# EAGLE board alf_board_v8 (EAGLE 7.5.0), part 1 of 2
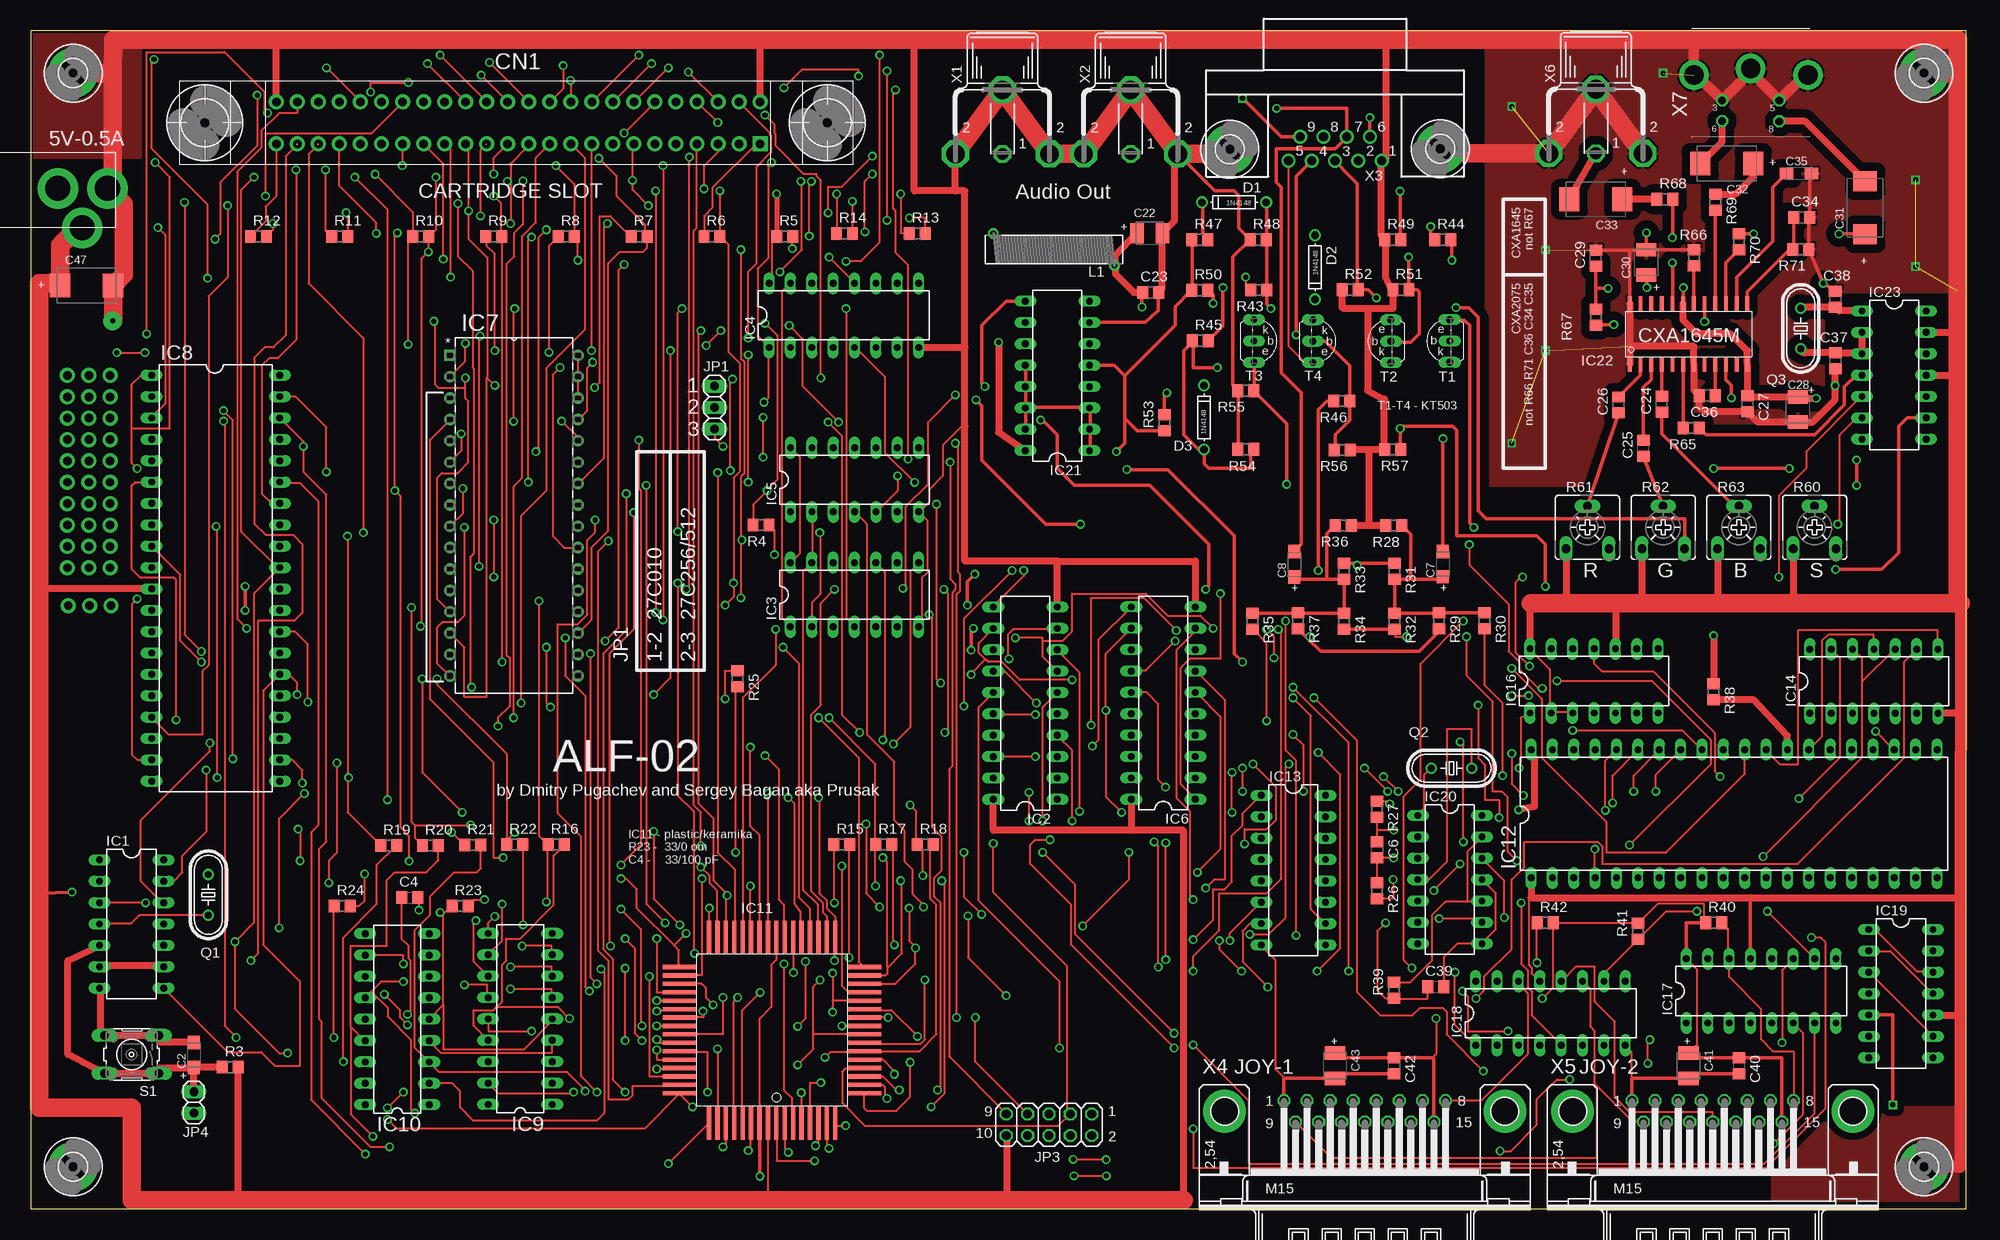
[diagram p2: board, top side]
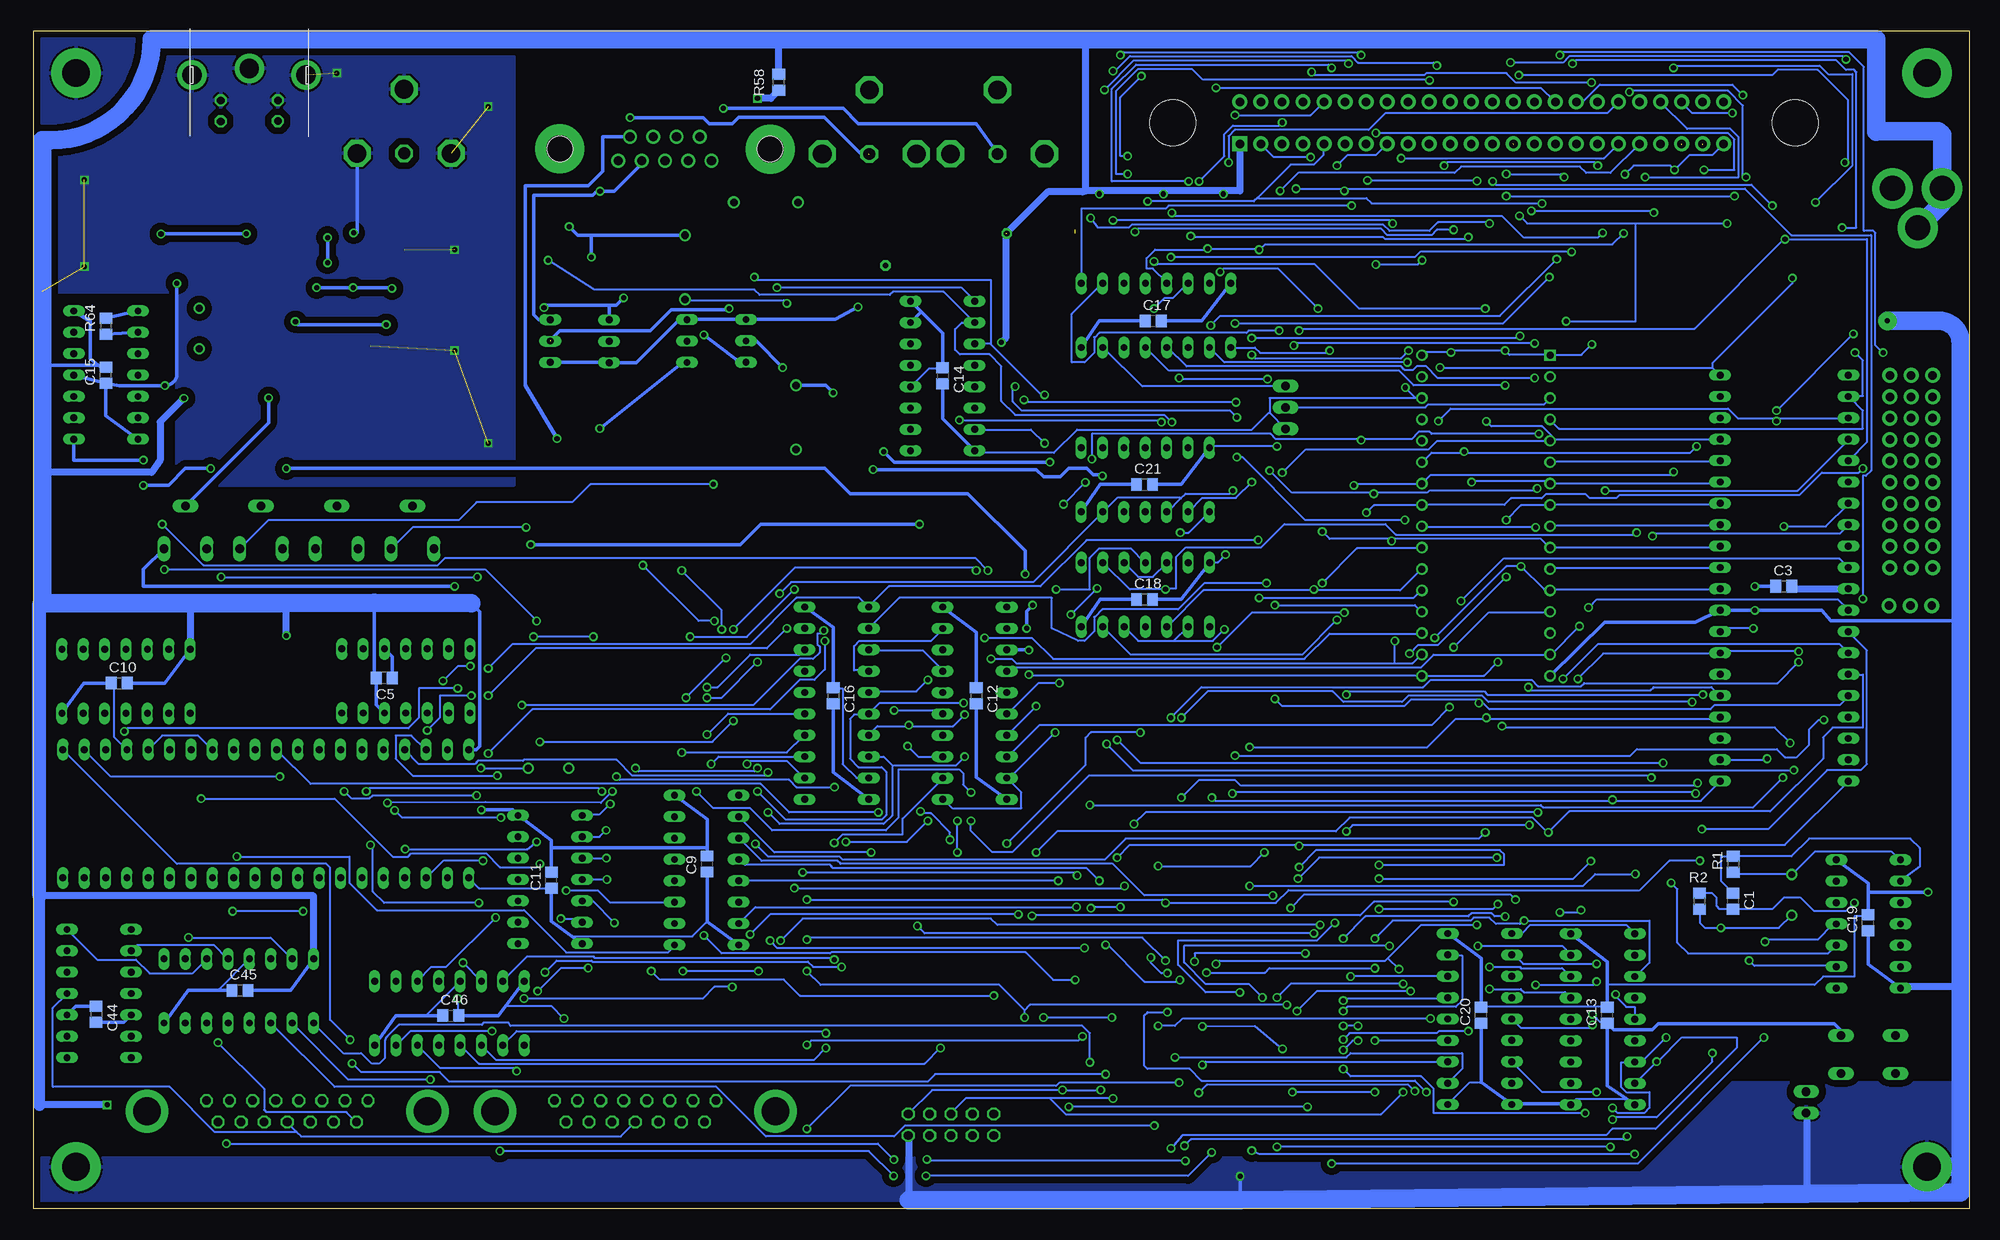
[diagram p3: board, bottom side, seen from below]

Size 230 x 140 mm. Coordinates in mm from the lower left corner, seen from the top.
Outline: 0,0 230,0 230,140 0,140 0,0
Copper layers (1*16): Top 0.035mm / dielectric 1.5mm / Bottom 0.035mm
Design rules "default *": minimum track width 10mil, minimum drill 24mil, track to track 8mil, track to pad 8mil, pad to pad 8mil, via to via 8mil, smd to smd 8mil, copper to edge 4mil, drill to drill 8mil, minimum pad ring 10mil, minimum via ring 8mil, stop-mask expansion 4mil, vias tented up to drill 24mil, thermal gap 10mil

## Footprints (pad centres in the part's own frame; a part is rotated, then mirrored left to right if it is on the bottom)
C0805 = smd 1.3 x 1.5: 1 -0.95,0; 2 0.95,0
SMC_A = smd 1.6 x 1.4: + -1.5,0; - 1.5,0
SMC_B = smd 1.6 x 2.4: + -1.5,0; - 1.5,0
SMC_D = smd 2.4 x 2.8: + -3.15,0; - 3.15,0
СНП15-48 = drill 1 pad 1.778 square: 1 29,-2.5 | drill 1 pad 1.778: 2 29,2.5; 3 26.5,-2.5; 4 26.5,2.5; 5 24,-2.5; 6 24,2.5; 7 21.5,-2.5; 8 21.5,2.5; 9 19,-2.5; 10 19,2.5; 11 16.5,-2.5; 12 16.5,2.5; 13 14,-2.5; 14 14,2.5; 15 11.5,-2.5; 16 11.5,2.5; 17 9,-2.5; 18 9,2.5; 19 6.5,-2.5; 20 6.5,2.5; 21 4,-2.5; 22 4,2.5; 23 1.5,-2.5; 24 1.5,2.5; 25 -1,-2.5; 26 -1,2.5; 27 -3.5,-2.5; 28 -3.5,2.5; 29 -6,-2.5; 30 -6,2.5; 31 -8.5,-2.5; 32 -8.5,2.5; 33 -11,-2.5; 34 -11,2.5; 35 -13.5,-2.5; 36 -13.5,2.5; 37 -16,-2.5; 38 -16,2.5; 39 -18.5,-2.5; 40 -18.5,2.5; 41 -21,-2.5; 42 -21,2.5; 43 -23.5,-2.5; 44 -23.5,2.5; 45 -26,-2.5; 46 -26,2.5; 47 -28.5,-2.5; 48 -28.5,2.5
DO-1N4148 = drill 0.9: A -3.81,0; C 3.81,0
3,3-PAD = drill 3.3 pad 5.842: B3,3 0,0
3,2-PAD = drill 3.2 pad 5.842: B3,2 0,0
DIL14 = drill 0.813 long: 1 -7.62,-3.81; 2 -5.08,-3.81; 3 -2.54,-3.81; 4 0,-3.81; 5 2.54,-3.81; 6 5.08,-3.81; 7 7.62,-3.81; 8 7.62,3.81; 9 5.08,3.81; 10 2.54,3.81; 11 0,3.81; 12 -2.54,3.81; 13 -5.08,3.81; 14 -7.62,3.81
DIL20 = drill 0.813 long: 1 -11.43,-3.81; 2 -8.89,-3.81; 3 -6.35,-3.81; 4 -3.81,-3.81; 5 -1.27,-3.81; 6 1.27,-3.81; 7 3.81,-3.81; 8 6.35,-3.81; 9 8.89,-3.81; 10 11.43,-3.81; 11 11.43,3.81; 12 8.89,3.81; 13 6.35,3.81; 14 3.81,3.81; 15 1.27,3.81; 16 -1.27,3.81; 17 -3.81,3.81; 18 -6.35,3.81; 19 -8.89,3.81; 20 -11.43,3.81
DIL16 = drill 0.813 long: 1 -8.89,-3.81; 2 -6.35,-3.81; 3 -3.81,-3.81; 4 -1.27,-3.81; 5 1.27,-3.81; 6 3.81,-3.81; 7 6.35,-3.81; 8 8.89,-3.81; 9 8.89,3.81; 10 6.35,3.81; 11 3.81,3.81; 12 1.27,3.81; 13 -1.27,3.81; 14 -3.81,3.81; 15 -6.35,3.81; 16 -8.89,3.81
DIP254P1524X482-32P = drill 0.838 square: 1 -15.24,38.1 | drill 0.838: 2 -15.24,35.56; 3 -15.24,33.02; 4 -15.24,30.48; 5 -15.24,27.94; 6 -15.24,25.4; 7 -15.24,22.86; 8 -15.24,20.32; 9 -15.24,17.78; 10 -15.24,15.24; 11 -15.24,12.7; 12 -15.24,10.16; 13 -15.24,7.62; 14 -15.24,5.08; 15 -15.24,2.54; 16 -15.24,0; 17 0,0; 18 0,2.54; 19 0,5.08; 20 0,7.62; 21 0,10.16; 22 0,12.7; 23 0,15.24; 24 0,17.78; 25 0,20.32; 26 0,22.86; 27 0,25.4; 28 0,27.94; 29 0,30.48; 30 0,33.02; 31 0,35.56; 32 0,38.1
DIL40 = drill 0.813 long: 1 -24.13,-7.62; 2 -21.59,-7.62; 3 -19.05,-7.62; 4 -16.51,-7.62; 5 -13.97,-7.62; 6 -11.43,-7.62; 7 -8.89,-7.62; 8 -6.35,-7.62; 9 -3.81,-7.62; 10 -1.27,-7.62; 11 1.27,-7.62; 12 3.81,-7.62; 13 6.35,-7.62; 14 8.89,-7.62; 15 11.43,-7.62; 16 13.97,-7.62; 17 16.51,-7.62; 18 19.05,-7.62; 19 21.59,-7.62; 20 24.13,-7.62; 21 24.13,7.62; 22 21.59,7.62; 23 19.05,7.62; 24 16.51,7.62; 25 13.97,7.62; 26 11.43,7.62; 27 8.89,7.62; 28 6.35,7.62; 29 3.81,7.62; 30 1.27,7.62; 31 -1.27,7.62; 32 -3.81,7.62; 33 -6.35,7.62; 34 -8.89,7.62; 35 -11.43,7.62; 36 -13.97,7.62; 37 -16.51,7.62; 38 -19.05,7.62; 39 -21.59,7.62; 40 -24.13,7.62
DIL18 = drill 0.813 long: 1 -10.16,-3.81; 2 -7.62,-3.81; 3 -5.08,-3.81; 4 -2.54,-3.81; 5 0,-3.81; 6 2.54,-3.81; 7 5.08,-3.81; 8 7.62,-3.81; 9 10.16,-3.81; 10 10.16,3.81; 11 7.62,3.81; 12 5.08,3.81; 13 2.54,3.81; 14 0,3.81; 15 -2.54,3.81; 16 -5.08,3.81; 17 -7.62,3.81; 18 -10.16,3.81
TQFP64 = smd 0.5 x 4: 1 -1.5,-13; 2 -0.5,-13; 3 0.5,-13; 4 1.5,-13; 5 2.5,-13; 6 3.5,-13; 7 4.5,-13; 8 5.5,-13; 25 5.5,9; 26 4.5,9; 27 3.5,9; 28 2.5,9; 29 1.5,9; 30 0.5,9; 31 -0.5,9; 32 -1.5,9; 33 -2.5,9; 34 -3.5,9; 35 -4.5,9; 36 -5.5,9; 37 -6.5,9; 38 -7.5,9; 39 -8.5,9; 40 -9.5,9; 57 -9.5,-13; 58 -8.5,-13; 59 -7.5,-13; 60 -6.5,-13; 61 -5.5,-13; 62 -4.5,-13; 63 -3.5,-13; 64 -2.5,-13 | smd 4 x 0.5: 9 9,-9.5; 10 9,-8.5; 11 9,-7.5; 12 9,-6.5; 13 9,-5.5; 14 9,-4.5; 15 9,-3.5; 16 9,-2.5; 17 9,-1.5; 18 9,-0.5; 19 9,0.5; 20 9,1.5; 21 9,2.5; 22 9,3.5; 23 9,4.5; 24 9,5.5; 41 -13,5.5; 42 -13,4.5; 43 -13,3.5; 44 -13,2.5; 45 -13,1.5; 46 -13,0.5; 47 -13,-0.5; 48 -13,-1.5; 49 -13,-2.5; 50 -13,-3.5; 51 -13,-4.5; 52 -13,-5.5; 53 -13,-6.5; 54 -13,-7.5; 55 -13,-8.5; 56 -13,-9.5
SOP24 = smd 0.45 x 1.8: 1 -6.97,-3.6; 2 -5.7,-3.6; 3 -4.43,-3.6; 4 -3.16,-3.6; 5 -1.89,-3.6; 6 -0.62,-3.6; 7 0.65,-3.6; 8 1.92,-3.6; 9 3.19,-3.6; 10 4.46,-3.6; 11 5.73,-3.6; 12 7,-3.6; 13 7,3.6; 14 5.73,3.6; 15 4.46,3.6; 16 3.19,3.6; 17 1.92,3.6; 18 0.65,3.6; 19 -0.62,3.6; 20 -1.89,3.6; 21 -3.16,3.6; 22 -4.43,3.6; 23 -5.7,3.6; 24 -6.97,3.6
PJ-102A = drill 3 pad 4.8: RING 0.1,-3.39; RING_SW -4.6,-6.29; TIP 0.1,-9.29
1X03 = drill 1.016 long: 1 -2.54,0; 2 0,0; 3 2.54,0
2X05 = drill 1.016 octagon: 1 -5.08,-1.27; 2 -5.08,1.27; 3 -2.54,-1.27; 4 -2.54,1.27; 5 0,-1.27; 6 0,1.27; 7 2.54,-1.27; 8 2.54,1.27; 9 5.08,-1.27; 10 5.08,1.27
1X02 = drill 1.016 long: 1 -1.27,0; 2 1.27,0
Z27/24 = drill 0.7 octagon: 1 7.2,-1.9; 2 -7.2,1.9
HC49/S = drill 0.813: 1 -2.413,0; 2 2.413,0
R0805 = smd 1.3 x 1.5: 1 -0.95,0; 2 0.95,0
CA6V = drill 1.016 long: A -2.54,-2.54; E 2.54,-2.54; S 0,2.54
B3F-10XX = drill 1.016 long: 1 -3.251,2.261; 2 3.251,2.261; 3 -3.251,-2.261; 4 3.251,-2.261
TO92-CBE = drill 0.813 long: B 0,0; C -2.54,0; E 2.54,0
5,5 = hole 5.5: 0,0
TOBU3 = drill 1.397 octagon: 1 0,-2.54 | drill 2.21 octagon: 2 5.588,-2.54; 2@1 -5.588,-2.54; 2@2 0,5.08
H5M09RA = drill 1.092: 1 -5.537,1.422; 2 -2.769,1.422; 3 0,1.422; 4 2.769,1.422; 5 5.537,1.422; 6 -4.153,-1.422; 7 -1.384,-1.422; 8 1.384,-1.422; 9 4.153,-1.422 | hole 3.048: -12.497,0; 12.497,0
M15HP = drill 1.016 octagon: 1 -9.601,1.27; 2 -6.858,1.27; 3 -4.115,1.27; 4 -1.372,1.27; 5 1.372,1.27; 6 4.115,1.27; 7 6.858,1.27; 8 9.601,1.27; 9 -8.23,-1.27; 10 -5.486,-1.27; 11 -2.743,-1.27; 12 0,-1.27; 13 2.743,-1.27; 14 5.486,-1.27; 15 8.23,-1.27 | drill 3.302 pad 5.08: G1 -16.662,0; G2 16.662,0
M_DIN4 = drill 0.9 pad 1.422 octagon: 3 -3.4,-3.75; 5 3.4,-3.75; 6 -3.4,-6.2; 8 3.4,-6.25 | drill 2.3 pad 3.5: SH1 6.8,-0.75; SH2 0,0.05; SH3 -6.75,-0.75

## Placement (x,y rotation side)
C1  68pF  [C0805]  28.06,36.58 270 bottom
C2  10uF 16V  [SMC_A]  19.36,18.29 90 top
C3  [C0805]  22,74 0 bottom
C4  33/100pF  [C0805]  45,37 0 top
C5  [C0805]  188.35,63.1 180 bottom
C6  68pF  [C0805]  159.99,42.66 270 top
C7  1uF  [SMC_A]  167.81,76.63 90 top
C8  1uF  [SMC_A]  150.16,76.61 90 top
C9  [C0805]  149.99,40.99 90 bottom
C10  [C0805]  219.86,62.49 0 bottom
C11  [C0805]  168.49,39.04 90 bottom
C12  [C0805]  118,61 270 bottom
C13  [C0805]  43,23 90 bottom
C14  [C0805]  122,99 270 bottom
C15  [C0805]  221.45,99.1 90 bottom
C16  [C0805]  135,61 270 bottom
C17  [C0805]  96.95,105.55 0 bottom
C18  [C0805]  98,72.45 0 bottom
C19  [C0805]  12,34 90 bottom
C20  [C0805]  58,23 90 bottom
C21  [C0805]  98,86.1 0 bottom
C22  100uF  [SMC_B]  132.98,115.97 0 top
C23  [C0805]  133.09,108.94 0 top
C24  [C0805]  193.85,95.65 90 top
C25  [C0805]  191.65,90.4 90 top
C26  [C0805]  188.7,95.55 90 top
C27  [C0805]  204,95.7 270 top
C28  47uF  [SMC_B]  210,95 270 top
C29  [C0805]  186,113 90 top
C30  47uF  [SMC_B]  192,112.5 90 top
C31  220uF  [SMC_D]  218,119 90 top
C32  220uF  [SMC_D]  201.55,124.25 180 top
C33  220uF  [SMC_D]  186,120 180 top
C34  [C0805]  210.45,117.85 0 top
C35  10uF  [SMC_A]  210.15,123.05 0 top
C36  [C0805]  199.25,96.65 180 top
C37  33  [C0805]  214.5,100.8 90 top
C38  33  [C0805]  214.45,108.1 270 top
C39  4n7  [C0805]  166.95,26.4 0 top
C40  [C0805]  203,17 270 top
C41  50uF  [SMC_B]  197,17 270 top
C42  [C0805]  162,17 270 top
C43  50uF  [SMC_B]  155,17 270 top
C44  [C0805]  222.61,23.11 270 bottom
C45  [C0805]  205.51,25.97 0 bottom
C46  [C0805]  180.46,22.97 0 bottom
C47  220uF  [SMC_D]  6.6,109.75 0 top
CN1  СНП15-48  [СНП15-48]  57.66,129.08 0 top
D1  1N4148  [DO-1N4148]  143,119.63 180 top
D2  1N4148  [DO-1N4148]  152.62,111.91 270 top
D3  1N4148  [DO-1N4148]  139.43,94.07 90 top
H1  MOUNT-PAD-ROUND3.3  [3,3-PAD]  5,135 0 top
H2  MOUNT-PAD-ROUND3.3  [3,3-PAD]  225,135 0 top
H3  MOUNT-PAD-ROUND3.3  [3,3-PAD]  225,5 0 top
H4  MOUNT-PAD-ROUND3.3  [3,3-PAD]  5,5 0 top
H5  MOUNT-PAD-ROUND3.2  [3,2-PAD]  142.5,125.95 0 top
H6  MOUNT-PAD-ROUND3.2  [3,2-PAD]  167.5,126 0 top
IC1  LS04/1533LN1  [DIL14]  11.95,33.86 270 top
IC2  ALS240 / 1533AP3  [DIL20]  118.18,60.1 90 top
IC3  ALS32/1533LL1  [DIL14]  97.88,73 0 top
IC4  ALS175/1533TM8  [DIL16]  96.62,106.2 0 top
IC5  ALS09/1533LI2  [DIL14]  97.9,86.65 0 top
IC6  LS245 / 555AP6  [DIL20]  134.58,60.11 90 top
IC7  27C010  [DIP254P1524X482-32P]  65.03,63.35 0 top
IC8  Z80A  [DIL40]  21.96,74.96 270 top
IC9  41464/RU11  [DIL18]  58.15,22.57 90 top
IC10  41464/RU11  [DIL18]  43.53,22.54 90 top
IC11  T34VG1  [TQFP64]  90.09,23.24 0 top
IC12  YM2149F / AY-3-8910  [DIL40]  202.43,46.96 0 top
IC13  ALS138/1533ID7  [DIL16]  150.05,40.26 270 top
IC14  ALS00/1533LA3  [DIL14]  219.05,62.7 0 top
IC16  ALS93/1533IE5  [DIL14]  185.79,62.75 0 top
IC17  74HC595  [DIL16]  205.65,25.9 0 top
IC18  74HC595  [DIL16]  180.61,23.25 0 top
IC19  7493 / 155IE5  [DIL14]  222.26,25.59 270 top
IC20  ALS04/1533LN1  [DIL14]  168.65,39.14 270 top
IC21  ALS251/1533KP15  [DIL16]  122,99 90 top
IC22  CXA1645  [SOP24]  197,104 0 top
IC23  74HCT04  [DIL14]  221.45,99.1 270 top
J1  2.1MMJACKTHM  [PJ-102A]  -0.2,121.2 90 top
JP1  [1X03]  81.25,95.25 270 top
JP3  V-TTL-OUT  [2X05]  121,10 180 top
JP4  RESET  [1X02]  19.35,12.65 270 top
L1  220 uH  [Z27/24]  121.59,114.03 180 top
Q1  8Mhz  [HC49/S]  21.08,37.33 270 top
Q2  14Mhz  [HC49/S]  168.84,52.38 0 top
Q3  4,433619Mhz  [HC49/S]  210.35,104.65 270 top
R1  510  [R0805]  28.02,40.95 90 bottom
R2  510  [R0805]  32.03,36.58 270 bottom
R3  100k  [R0805]  23.69,16.84 0 top
R4  1.6k  [R0805]  86.77,81.28 180 top
R5  2.2k  [R0805]  89.59,115.59 0 top
R6  2.2k  [R0805]  80.94,115.59 0 top
R7  2.2k  [R0805]  72.29,115.59 0 top
R8  2.2k  [R0805]  63.64,115.59 0 top
R9  2.2k  [R0805]  54.99,115.59 0 top
R10  2.2k  [R0805]  46.34,115.59 0 top
R11  2.2k  [R0805]  36.69,115.59 0 top
R12  2.2k  [R0805]  27.04,115.59 0 top
R13  10k  [R0805]  105.34,115.94 0 top
R14  10k  [R0805]  96.69,115.94 0 top
R15  1k  [R0805]  96.39,43.29 0 top
R16  1k  [R0805]  62.44,43.29 0 top
R17  1k  [R0805]  101.36,43.29 0 top
R18  1k  [R0805]  106.29,43.29 0 top
R19  1k  [R0805]  42.5,43.19 0 top
R20  1k  [R0805]  47.48,43.19 0 top
R21  1k  [R0805]  52.51,43.24 0 top
R22  1k  [R0805]  57.49,43.29 0 top
R23  33/0  [R0805]  51,36 0 top
R24  33  [R0805]  37,36 0 top
R25  300  [R0805]  83.99,63.02 270 top
R26  510  [R0805]  159.97,37.81 270 top
R27  510  [R0805]  159.97,47.51 270 top
R28  2.2k  [R0805]  161.99,81.22 0 top
R29  1k  [R0805]  167.35,69.9 270 top
R30  1k  [R0805]  172.77,69.91 270 top
R31  15k  [R0805]  162.07,75.81 270 top
R32  2.2k  [R0805]  162.07,69.86 270 top
R33  15k  [R0805]  156.07,75.81 270 top
R34  2.2k  [R0805]  156.07,69.86 270 top
R35  1k  [R0805]  145.17,69.86 270 top
R36  2.2k  [R0805]  155.96,81.23 180 top
R37  1k  [R0805]  150.6,69.9 270 top
R38  1k  [R0805]  199.99,61.46 270 top
R39  1.5k  [R0805]  162,26 90 top
R40  10k  [R0805]  200,34 0 top
R41  1k  [R0805]  191.01,32.99 90 top
R42  10k  [R0805]  180,34 0 top
R43  1k  [R0805]  145.91,109.21 180 top
R44  1k  [R0805]  167.79,115.19 0 top
R45  1k  [R0805]  138.99,103.19 0 top
R46  1.5k  [R0805]  155.81,96.01 180 top
R47  3k3  [R0805]  138.94,115.19 0 top
R48  3k3  [R0805]  145.89,115.19 0 top
R49  200  [R0805]  161.84,115.19 0 top
R50  3k3  [R0805]  138.94,109.19 0 top
R51  3k3  [R0805]  162.84,109.24 0 top
R52  200  [R0805]  156.79,109.24 0 top
R53  3k3  [R0805]  134.71,93.44 90 top
R54  3k3  [R0805]  144.39,90.29 0 top
R55  200  [R0805]  144.39,97.24 0 top
R56  2k  [R0805]  155.86,90.21 180 top
R57  200  [R0805]  161.84,90.24 0 top
R58  100  [R0805]  141.47,133.89 90 bottom
R60  [CA6V]  212,81 0 top
R61  [CA6V]  185,81 0 top
R62  [CA6V]  194,81 0 top
R63  [CA6V]  203,81 0 top
R64  4.7M  [R0805]  221.45,104.9 90 bottom
R65  1.6k  [R0805]  197.35,92.8 180 top
R66  16k  [R0805]  197.65,113.05 90 top
R67  2.4k  [R0805]  186,106 270 top
R68  75  [R0805]  194.2,120 0 top
R69  75  [R0805]  200.2,119.65 270 top
R70  75  [R0805]  203,114.95 270 top
R71  47k  [R0805]  210.35,114.05 180 top
S1  RESET  [B3F-10XX]  11.97,18.35 180 top
T1  [TO92-CBE]  168.63,103.15 90 top
T2  [TO92-CBE]  161.63,103.12 90 top
T3  [TO92-CBE]  145.37,103.16 270 top
T4  [TO92-CBE]  152.37,103.14 270 top
U$2  [5,5]  20.65,129.1 0 top
U$3  [5,5]  94.65,129.1 0 top
X1  RCA_L  [TOBU3]  115.47,127.93 0 top
X2  RCA_R  [TOBU3]  130.71,127.93 0 top
X3  RGB-OUT  [H5M09RA]  155,126 180 top
X4  JOY-1  [M15HP]  158.53,11.59 0 top
X5  JOY-2  [M15HP]  199.89,11.59 0 top
X6  Video  [TOBU3]  186,128 0 top
X7  s-video  [M_DIN4]  204.4,135.5 0 top

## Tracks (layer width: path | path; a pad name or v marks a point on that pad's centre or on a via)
1IC8  (via drill 0.61)
  Top 0.254: v141.38,73.12 141.38,65.38 137.75,65.38 136.62,64.25 136.62,50.5 138.38,48.75 IC6.1 | v49.88,110.75 49.88,125.88 49.25,126.5 CN1.31 | v87.25,105.25 88.75,103.75 88.75,86.75 87.5,85.5 v87.5,85.38 85.82,83.69 R4.2
  Bottom 0.254: v87.5,85.38 87.88,85 93.12,85 93.69,84.44 | 93.69,84.44 95.25,82.88 IC5.3 | 93.69,84.44 93.75,84.5 101.25,84.5 102.88,82.88 IC5.6 103,82.75 111.25,74.5 140,74.5 v141.38,73.12 | v49.88,110.75 55.38,105.25 v87.25,105.25
8M  (via drill 0.61)
  Top 0.254: IC1.4 8.25,33.88 11.88,33.88 12.88,34.88 21,34.88 Q1.2 | v87.55,49.38 87.55,32.5 87.5,32.25 IC11.33 | v32.5,49.38 29.5,46.38 v29.5,33.4
  Bottom 0.254: v87.55,49.38 87.12,49.5 32.62,49.5 v32.5,49.38 | R2.2 32,35.6 32,34 31.4,33.4 v29.5,33.4 22.6,33.4 Q1.2
+5V  (via drill 0.6, 0.6 pad 0.25, 0.61)  (1 unrouted)
  Top 0.254: IC3.14 90.38,76.88 91.38,77.88 91.38,89.38 90.38,90.38 IC5.14 | v67,97.62 67.62,98.25 67.62,118 68.88,118 71.25,115.62 R7.1 | v82.25,90.62 81.25,91.62 JP1.3 | R12.1 27.88,117.38 27.88,119.12 29.12,120.38 29.12,126.5 CN1.47 | v35,123.5 35,116.25 35.62,115.62 R11.1 | 45.38,115.62 R10.1 | v55.12,102 55.12,113.5 54.12,114.5 54.12,115.5 R9.1 | 62.62,115.5 R8.1 61.58,114.47 v61.58,101.8 | IC7.32 65,101.38 65,99 IC7.31 65,98.88 65,96.38 IC7.30 | 45.5,115.5 R10.1 | IC4.16 87.75,110.12 88.12,110.5 88.12,115 88.62,115.5 R5.1 88.62,115.62 | 24.62,16.75 R3.2 | 200,62.5 R38.1 | 80,115.62 R6.1 80,118 81,119 81,121.38 86.12,126.5 86.62,126.5 CN1.1 | v95.75,120.62 95.75,116 R14.1 | v103.38,120.62 103.38,116 R13.1 | 87.62,1 87.62,10.12 IC11.64 | R40.1 198.88,34.12 198.88,36.25 193.38,36.25 191.12,34 R41.2 191,34 R42.2 180.88,34 180.88,26.25 v179.62,25 | v167,22.62 167,18.38 166.75,18.12 166.75,17.95 | v88.38,77.75 88.38,80.62 R4.1 | v44.83,102.75 44.83,115.03 R10.1 | v40.9,122.97 45.39,118.48 R10.1 | C41.+ 198.05,19.55 198.05,28.42 IC17.16
  Top 0.406: R67.1 186,109.4 | 186,109.4 C29.1 | C30.+ 192.05,111 v192.05,109.5 | v187.45,109.4 186,109.4 | v196.4,109.5 196.38,109.5 IC22.19 | C27.1 204.15,96.5 | R40.1 196.76,34 IC17.16 | C43.+ 155,17.95 C42.1 166.75,17.95 166.76,17.95 X4.15 | C41.+ 197,17.95 C40.1 208.12,17.95 X5.15 | JP3.10 116,8.73 | 1,73.69 1,74 | v4.88,37.65 1,37.5 | IC19.5 221.3,23.05 v221.3,12.35
  Top 0.61: v88.62,120.62 88.62,115.62
  Top 0.813: IC22.19 196.38,105.62 198,104 202,104 204,102 IC22.12 C27.1 | 204.15,96.5 C28.+ 210.15,96.35 v212.2,96.35 | 137,1 137,45 130.77,45 | 130.77,45 114.4,45 114.4,48.67 IC2.20 | IC6.20 130.77,45 | 116,8.73 116,1 | IC8.11 1,73.69 | 24.62,1 24.62,16.75 | v200,68.12 200,62.5 | v176.82,47.42 178.7,47.8 178.7,53.55 IC12.40 | v115,103 115,92.3 IC21.16 | 0.99,47 1,47
  Top 2.184: 137,1 116,1 87.62,1 24.62,1 12,1 12,12 1,12 1,37.5 1,47 1,74 1,110 3.45,110 C47.+ 3.45,114.55 5.5,116.6 J1.RING_SW
  Bottom 0.254: v88.38,77.75 89.25,76.88 90.12,76.88 IC3.14 | 65.81,96.44 65.75,96.38 65.12,96.38 IC7.30 | 65.81,96.44 v67,97.62 | 83.12,94.62 81.25,92.75 JP1.3 | 83.12,94.62 83.12,96.38 65.88,96.38 65.81,96.44 | v82.25,90.62 90,90.62 90.12,90.5 IC5.14 | CN1.47 29.25,126.5 30.5,125.25 33.25,125.25 v35,123.5 35.5,124 39.88,124 v40.9,122.97 | C20.2 57.88,24 43.12,24 C13.2 | v95.75,120.62 95.75,121 | v103.38,120.62 103.38,121 | 114.38,116 L1.1 | v88.62,120.62 88.62,121 | 189.57,63.3 C5.2 | v179.62,25 179.62,23.12 C46.2 | 43,26.62 18.35,26.62 17.32,27.6 13.62,27.6 13.62,34.75 12,34.75 C19.2 | 172.62,46.88 IC20.14 | v167,22.62 168.5,24.12 173.75,24.12 173.87,24.21 | 83.12,94.62 83.25,94.62 85.25,92.62 106,92.62 108.78,89.85 117.93,89.85 arc90 IC21.16 118,90.12 | v44.83,102.75 46.08,101.5 49.75,101.5 IC7.1 49.88,101.5 54.62,101.5 v55.12,102 61.38,102 v61.58,101.8 64.68,101.8 IC7.32
  Bottom 0.406: C19.2 12,37.65 | 12,37.65 12,38.72 IC1.14 | C13.2 43,26.62 43,29.36 IC10.9 | C20.2 58,29.77 IC9.9 | C12.2 118,51.3 IC2.20 | C16.2 135,51.91 IC6.20 | C18.2 93.62,72.45 IC3.14 | C21.2 93.64,86.1 IC5.14 | C17.2 91.19,105.55 IC4.16 | C14.2 122,93.92 IC21.16 | C9.2 149.99,42.9 | 149.99,42.9 149.99,46.28 IC13.16 | C46.2 174.81,22.97 173.87,24.21 IC18.16 | C45.2 199.5,25.97 IC17.16 | C44.2 219.34,22.16 IC19.5 | C10.2 214.45,62.49 IC14.14 211.35,66.59 | C5.2 189.3,59.91 IC16.5 | C11.2 168.49,42.9 | 168.49,42.9 168.49,43.79 IC20.14 | IC23.14 223.3,105.51 223.3,101.05 222.05,100.05 C15.2 221.7,100.3 229,100.3 | v187.45,109.4 187.45,109.5 v192.05,109.5 v196.4,109.5 | 178,72 177,71 177,55 177.42,54.58 IC12.40 | 149.99,42.9 168.49,42.9 | 189.57,72.05 189.57,63.3 | v4.88,37.65 12,37.65 | 172.62,46.88 173.07,47.42 v176.82,47.42 | 141.47,138.47 142,139
  Bottom 0.813: 211.35,66.59 211.35,72 | v212.2,96.35 215,93.55 215,89 216,87.55 229,87.55 | CN1.1 86.66,121 88.62,121 95.75,121 103.38,121 105,121 | 105,121 105,139 | IC17.16 196.76,37.2 229.35,37.2 | v200,68.12 200,72 | 114.38,116 109.5,120.88 105.38,120.88 105,121 | v221.3,12.35 229.35,12.35 | C3.2 20.74,73.69 IC8.11 | R58.2 141.47,138.47 | 114.5,115.88 114.5,103.5 v115,103
  Bottom 1.422: 229.35,12.35 229.35,37.2
  Bottom 1.676: 229.35,37.2 229.35,72 229,72
  Bottom 2.184: 178,72 189.57,72.05 200,72 211.35,72 229,72 229,87.55 229,100.3 229,127 228,127 arc-90 216,139 142,139 105,139 11,139 11,128 10.9,128.1 3.65,128.1 3.19,127.64 J1.RING 3.19,119.5 J1.RING_SW
/BUSRQ  (via drill 0.61)
  Top 0.254: 97.62,116 R14.2 97.62,115.95 v97.62,119.75 | v50.75,119.5 50.75,113.25 52.5,111.5 52.5,100 52.65,99.85 52.65,77.9 52.2,77.45 52.2,62.17 v52.38,62
  Bottom 0.254: v97.62,119.75 85,119.75 84.56,120.19 | 84.56,120.19 80.62,124.12 77.88,124.12 76.75,125.25 76.75,126.5 CN1.9 | v52.38,62 52,61.62 37.88,61.62 37.5,62 30.62,62 29.62,61 IC8.25 | v50.75,119.5 71,119.5 71.62,120.12 84.5,120.12 84.56,120.19
/CAS  (via drill 0.61)
  Top 0.254: v85.5,38.38 85.5,32.25 IC11.35 | R24.2 39,36 39.65,36.65 v39.65,39.8
  Bottom 0.254: v85.5,38.38 45.88,38.38 44.45,39.8 v39.65,39.8
/CE  (via drill 0.61)
  Top 0.254: v93.75,80.38 93.88,80.25 93.88,73.12 92.88,72.12 92.88,69.25 IC3.2 | v88.5,68.88 88.5,64.62 84.62,60.75 84.62,32.25 IC11.36
  Bottom 0.254: 94.44,67.56 94.5,67.5 98.75,67.5 100.38,69.12 IC3.5 | 94.44,67.56 92.88,69.12 IC3.2 | v93.75,80.38 92.75,80.38 90.38,82.75 IC5.1 | v88.5,68.88 89.88,67.5 94.38,67.5 94.44,67.56
/INT  (via drill 0.61)
  Top 0.254: v82.5,60.62 82.5,63.97 R25.1 83.88,63.88 | v58.25,60.12 58.25,82.38 61.25,85.38 61.25,99.9 65.88,104.53 65.88,124.88 64.25,126.5 CN1.19
  Bottom 0.254: v82.5,60.62 81.62,59.75 67.12,59.75 66.38,60.5 58.25,60.5 | 58.25,60.5 58.12,60.5 57,59.38 30.75,59.38 30.25,59.88 15.38,59.88 14.38,60.88 IC8.16 | 58.25,60.5 v58.25,60.12
/IORQ  (via drill 0.61)
  Top 0.254: v103.38,39 103.5,38.88 103.5,30.38 101.81,28.69 | 101.81,28.69 101.81,28.01 101.55,27.75 99.12,27.75 IC11.23 | v101.25,41.75 101.75,41.25 101.75,28.75 101.81,28.69 | v79.62,43.12 79.62,47.12 78.75,48 78.75,116.25 79.12,116.62 79.12,126.5 CN1.7
  Bottom 0.254: v103.38,39 104.88,40.5 135,40.5 135.38,40.88 145.5,40.88 146.12,41.5 IC13.4 | 79.62,43.25 99.75,43.25 v101.25,41.75 | 79.62,43.25 21.88,43.25 14.38,50.75 IC8.20 | v79.62,43.12 79.62,43.25
/M1  (via drill 0.61)
  Top 0.254: v142.5,31.88 142.5,32.75 146.12,36.38 IC13.6 | IC11.22 99.12,26.75 102.75,26.75 105.12,29.12 v105.12,31 105.12,31.12 104.38,31.88 v104.38,35.75 | v20.25,66.25 18.25,68.25 v18.25,119.62 | v35.12,135.62 39.12,131.62 CN1.40 | v100.88,35.88 99.25,37.5 v99.25,45.75 | v51.25,47.12 46.5,51.88 v46.5,63
  Bottom 0.254: v142.5,31.88 141.62,31 v105.12,31 | v20.25,66.25 29.38,66.25 29.5,66.12 IC8.27 29.62,66 43.5,66 v46.5,63 | v18.25,119.62 13.88,124 13.88,134.88 16.75,134.88 17.75,135.88 34.88,135.88 v35.12,135.62 | v104.38,35.75 104.25,35.88 v100.88,35.88 | v99.25,45.75 97.88,47.12 v51.25,47.12
/MREQ  (via drill 0.61)
  Top 0.254: v89.38,66.75 91.25,64.88 91.25,37.05 92.55,35.75 92.55,34.15 92.6,34.15 92.6,34.1 92.5,32.25 IC11.28 | v74.25,121 v74.25,70.88 | v80,121.25 80,124 81.66,125.66 CN1.5 | v12.62,72.5 12,71.88 12,54 12.63,53.37 IC8.19
  Bottom 0.254: v12.62,72.5 12.62,87.12 12.25,87.12 11.62,87.75 11.62,115.75 21.12,115.75 26.62,121.25 74.25,121.25 | v80,121.25 74.25,121.25 | v89.38,66.75 85.25,70.88 v74.25,70.88 | v74.25,121 74.25,121.25
/NMI  (via drill 0.61)  (1 unrouted)
  Top 0.254: 57,122.12 57,124.25 59.12,126.38 59.12,126.5 CN1.23 | 57,122.12 v57,117.12 | v23.38,119.25 23.38,110.75 21.12,108.5 21.12,64.62 20.38,63.88 20.38,56.38 16.38,56.38 14.38,58.38 IC8.17 | 57,122.12 v56.62,122.12 | 106.3,116.35 106.3,117.78 v104.4,117.78
  Bottom 0.254: v104.4,117.78 103.5,116.62 99.88,116.62 99.5,117 69.62,117 68.88,116.25 64.12,116.25 63.12,117.25 57.12,117.25 v57,117.12 | v23.38,119.25 25.88,121.75 56.25,121.75 v56.62,122.12
/RAS  (via drill 0.61)
  Top 0.254: v80.62,35.75 80.62,32.25 IC11.40 | R23.2 52.7,36.75 v53.9,36.75
  Bottom 0.254: v80.62,35.75 79,37.38 54.52,37.38 v53.9,36.75
/RD  (via drill 0.61)
  Top 0.254: v90,48.88 90.75,48.12 90.75,36.27 91.5,35.3 91.5,32.25 IC11.29 | v42.38,48.62 42.38,118.75 v38.5,122.62
  Bottom 0.254: 42.38,48.5 89.62,48.5 v90,48.88 | 42.38,48.5 31.88,48.5 29.62,50.75 IC8.21 | v38.5,122.62 27.38,122.62 27.38,127.38 28.38,128.38 33.5,128.38 36.62,131.5 CN1.42 | v42.38,48.62 42.38,48.5
/RES  (via drill 0.61)
  Top 0.254: IC1.8 23.38,18.62 27.38,18.62 29,17 32,17 32,27 27.6,31.4 27.6,61.6 29.5,63.5 IC8.26 30.62,63.53 31.62,62.52 v31.62,61.12 | v88,124.38 87.62,124 87.62,113 86.38,111.75 86.38,103.75 87.62,102.5 IC4.1 87.62,102.38 87.62,96.38 v87.12,95.88 | v219.25,56.75 221.38,54.62 IC12.23 | v179.62,61.88 179.12,61.88 176.88,64.12 176.88,65 175.62,66.25 175.62,71.88 170.95,76.55 v170.95,78.95 | v74,61.12 76,63.12 v76,102
  Top 0.406: v112.33,96.15 113,95.47 113,89 120.62,81.38 v124.75,81.38
  Bottom 0.254: v88,124.38 88,127.5 87.25,128.25 71.38,128.25 69.38,130.25 43,130.25 41.75,131.5 CN1.38 | v219.25,56.75 218.88,57.12 185.5,57.12 184.25,58.38 184.25,61.88 v179.62,61.88 | v112.33,96.15 112,95.88 v87.12,95.88 | v31.62,61.12 57.25,61.12 57.62,61.5 73.62,61.5 v74,61.12 | v76,102 76.25,101.75 84.25,101.75 84.88,102.38 87.62,102.38 IC4.1
  Bottom 0.406: v124.75,81.38 143.62,81.38 146.05,78.95 v170.95,78.95
/RFSH  (via drill 0.61)
  Top 0.254: v25.62,69 24.5,70.12 24.5,123.25 27.38,126.12 27.38,128.12 29.5,130.25 31.62,130.25 31.62,131.5 CN1.46 | v93.62,58.38 98.38,53.62 98.38,29.38 99,28.75 IC11.24 | v32.9,60.25 32.9,67.1 31.39,68.61 IC8.28
  Bottom 0.254: v25.62,69 29.12,69 29.5,68.62 IC8.28 | v93.62,58.38 90.5,61.5 75.62,61.5 74.38,60.25 67.38,60.25 66.62,61 57.88,61 57.12,60.25 v32.9,60.25
/ROM  (via drill 0.61)
  Top 0.254: v78.25,125 78.25,74 v77.88,73.62
  Bottom 0.254: 77.88,73.5 67.62,73.5 65.12,76 IC7.22 | 77.88,73.5 91,73.5 95.25,69.25 IC3.3 | v78.25,125 82.62,125 84.12,126.5 CN1.3 | v77.88,73.62 77.88,73.5
/ROMC  (via drill 0.61)
  Top 0.254: v75.12,124 v75.12,70
  Bottom 0.254: v75.12,70 79.25,65.88 99.62,65.88 102.88,69.12 IC3.6 | v75.12,124 73.88,125.25 70.5,125.25 69.25,126.5 CN1.15
/SSRD  (via drill 0.61)
  Top 0.254: IC5.2 92.88,82.75 92.88,76.88 IC3.13 92.75,76.75 91.75,75.75 91.75,37.95 93.5,36.2 93.5,32.25 IC11.27 | v66.62,102 66.62,126.5 CN1.17 | v85.25,86.38 v85.25,101.5
  Bottom 0.254: v66.62,102 67.5,101.12 84.88,101.12 v85.25,101.5 | v85.25,86.38 87.12,84.5 91.12,84.5 92.75,82.88 IC5.2
/SSWR  (via drill 0.61)  (1 unrouted)
  Top 0.254: v95.5,73.62 93.88,72 93.88,59.88 92.75,58.75 92.75,37.75 94.12,36.38 94.12,35.27 94.6,34.8 IC11.26 94.5,32.25 | 34.12,126.5 33,125.38 33,110 39.5,103.5 v39.5,80.38
  Bottom 0.254: IC3.9 102.88,76.75 99.75,73.62 v95.5,73.62 95.5,73.75 94.25,73.75 94.25,77.5 93.12,78.62 84.12,78.62 81.38,81.38 69.38,81.38 68.12,80.12 39.5,80.12 v39.5,80.38
/WAIT  (via drill 0.61)
  Top 0.254: IC11.34 86.5,32.25 86.62,31.57 86.6,32.38 86.6,44.4 85.5,45.5 v85.5,54.88 | v57.38,58.38 57.38,85.88 58.38,86.88 58.38,115.62 60,117.25 60,124.92 CN1.21
  Bottom 0.254: 57.38,58.25 61,58.25 64.38,54.88 v85.5,54.88 | 57.38,58.25 29.75,58.25 29.62,58.38 IC8.24 | v57.38,58.38 57.38,58.25
/WE  (via drill 0.61)
  Top 0.254: IC9.4 61.88,20 61.88,18.5 48.75,18.5 47.34,19.91 IC10.4 | v70.62,20 v70.62,28.6 | IC11.30 90.62,32.12 v90.62,28.07
  Bottom 0.254: v70.62,20 62,20 IC9.4 | v90.62,28.07 83.67,28.07 83.15,28.6 v70.62,28.6
/WR  (via drill 0.61)
  Top 0.254: v138.12,32 140.5,34.38 140.5,38 141.88,38 142.75,38.88 142.75,44.38 144,45.62 144,47 146.12,49.12 IC13.1 | v95.5,29.5 95.5,32.12 IC11.25 | v93.62,48.88 93.78,48.73 93.78,37.48 94.62,36.62 94.62,35.7 95.59,34.73 IC11.25 | 95.5,32.25 IC11.25 | v28.12,130.25 27.75,130.62 27.75,132.75 23,137.5 13.75,137.5 v13.75,104 | v22.88,94.88 24,93.75 v24,53.5 | v32.25,50.62 32.25,52.15 31.03,53.37 IC8.22
  Bottom 0.254: v138.12,32 137.88,32.25 98.25,32.25 v95.5,29.5 | v32.25,50.62 32.5,50.38 86.62,50.38 87.25,51 91.5,51 v93.62,48.88 | v28.12,130.25 32.88,130.25 34.12,131.5 CN1.44 | v22.88,94.88 v13.75,104 | v24,53.5 24.12,53.38 29.5,53.38 IC8.22
A0  (via drill 0.61)
  Top 0.254: v85.25,103.5 85.25,111.38 86.25,112.38 86.25,123.88 88,125.62 88,127.5 87.88,127.62 87.88,127.88 84.25,131.5 CN1.4 | v53.38,103.75 53.25,103.62 v53.25,76.38 | v79.88,23.5 79.88,22.75 77.12,22.75 IC11.47 | v66.38,25.88 65.88,26.38 65.88,61 63.5,63.38 v63.5,67.88
  Bottom 0.254: IC8.30 29.62,73.62 49.75,73.62 IC7.12 49.88,73.62 50.5,73.62 v53.25,76.38 55,76.38 v63.5,67.88 | v85.25,103.5 53.62,103.5 v53.38,103.75 | v79.88,23.5 77.5,25.88 v66.38,25.88
A1  (via drill 0.61)
  Top 0.254: v108.25,39 108.62,38.62 108.62,13.75 v107,12.12 | v78.62,12.12 77.12,13.62 IC11.56 77,13.62 72.92,9.55 43.5,9.55 42.42,10.62 v42.38,10.62 | v78.12,135.12 81.62,131.62 CN1.6 | v44.88,133.88 40.38,133.88 v40.38,132.75 | v26.5,122.62 25,121.12 25,80.5 29.38,76.12 IC8.31 29.5,76.12 26.5,73.12 26.5,34 v24.25,31.75 24.25,23.75 29.5,18.5 v30.5,18.5
  Bottom 0.254: v108.25,39 146.12,39 IC13.5 | v78.62,12.12 v107,12.12 | IC7.11 49.75,76.12 29.62,76.12 IC8.31 | v78.12,135.12 77.75,134.75 64.75,134.75 64.5,135 55,135 53.88,133.88 v44.88,133.88 | v40.38,132.75 40.25,132.88 28.62,132.88 26.88,131.12 26.88,122.62 v26.5,122.62 | v42.38,10.62 42.12,10.88 37.12,10.88 30.5,17.5 v30.5,18.5 | v24.25,31.75 24,32 18,32 16.25,33.75 15.87,33.75 IC1.11
A2  (via drill 0.61)
  Top 0.254: v81.62,129.12 79.25,131.5 CN1.8 | v91.5,122.12 91.62,122 91.62,114 v89,111.38 | v77.38,107 76.88,106.5 v76.88,80.5 | v68.62,79.38 67.38,78.12 67.38,30.75 68.62,29.5 68.62,13 71,13 71.5,13.5 71.5,14.62 77,14.62 IC11.55
  Bottom 0.254: IC8.32 29.62,78.75 29.75,78.62 49.75,78.62 IC7.10 49.88,78.62 50.88,79.62 68.62,79.62 | v81.62,129.12 82,128.75 87.5,128.75 88.5,127.75 88.5,125.12 v91.5,122.12 | v89,111.38 88.62,111.75 82.12,111.75 v77.38,107 | v76.88,80.5 76,79.62 68.62,79.62 | v68.62,79.38 68.62,79.62
A3  (via drill 0.61)
  Top 0.254: v87.25,130 88.38,128.88 88.38,127.88 88.5,127.75 88.5,126.38 91.88,123 93.38,123 93.38,122.75 93.88,122.25 v93.88,98.75 | v83.38,98.62 83.12,98.38 v83.12,87.75 | v80.42,13.88 80.42,18.62 77.12,18.62 IC11.51 | v70.62,13.88 69.12,15.38 69.12,29.75 68,30.88 68,66 70.75,68.75 v70.75,85 | IC7.9 51.35,82.69 51.35,85.62 v51.33,85.62
  Bottom 0.254: IC8.33 29.62,81.25 49.75,81.25 IC7.9 | v87.25,130 78.25,130 76.75,131.5 CN1.10 | v93.88,98.75 93.75,98.62 v83.38,98.62 | v83.12,87.75 80.5,85.12 70.75,85.12 | 70.75,85.12 64.38,85.12 64.1,85.4 51.55,85.4 v51.33,85.62 | v70.62,13.88 v80.42,13.88 | v70.75,85 70.75,85.12
A4  (via drill 0.61)
  Top 0.254: v70.5,127.88 74.12,131.5 CN1.12 | v82.25,25.12 82.25,20.75 77.12,20.75 IC11.49 | v67.25,26.75 66.5,27.5 v66.5,66 | v55,81.88 v55,75.12 | IC8.34 28.6,83.85 27.45,85 27.45,100.25 28.3,101.1 29.3,101.1 31.5,103.3 v31.5,123.5
  Bottom 0.254: IC8.34 29.62,83.75 49.75,83.75 IC7.8 49.88,83.62 53.25,83.62 v55,81.88 | v70.5,127.88 28.62,127.88 27.88,127.12 27.88,123.5 v31.5,123.5 | v82.25,25.12 80.62,26.75 v67.25,26.75 | v66.5,66 65.5,67 63.12,67 v55,75.12
A5  (via drill 0.61)
  Top 0.254: v75.75,135.62 71.75,131.62 CN1.14 | v92.75,122.12 92.5,121.88 v92.5,115.62 | v59.5,115.5 59.12,115.12 v59.12,86.38 | v39.75,6.5 33.3,12.95 33.3,44.75 34.15,45.6 34.15,84.1 32,86.25 29.72,86.25 IC8.35 | IC11.62 85.5,10.12 85.6,9.93 85.55,9.88 85.55,7.22 v85.25,6.92
  Bottom 0.254: v75.75,135.62 76.12,136 99,136 101.88,133.12 101.88,122.12 v92.75,122.12 | v92.5,115.62 92.38,115.5 69.62,115.5 69.38,115.25 59.75,115.25 v59.5,115.5 | v59.12,86.38 59,86.5 50.12,86.5 49.88,86.25 IC7.7 49.75,86.25 29.75,86.25 29.62,86.38 29.59,86.38 IC8.35 | v85.25,6.92 84.38,6.5 v39.75,6.5
A6  (via drill 0.61)
  Top 0.254: v73.75,136.12 69.25,131.62 CN1.16 | v102.75,133 102.5,132.75 102.5,118.9 102.75,118.65 102.75,113.67 104.25,112.17 v104.25,89.12 | v79.62,40.62 80.62,39.62 80.62,38.75 81.5,37.88 81.5,32.25 IC11.39 | v70.12,40.88 72.5,43.25 72.5,85.38 72.25,85.62 v72.25,91.38 | v51.12,92.12 51.12,90.08 IC7.6
  Bottom 0.254: IC8.36 29.62,88.88 49.62,88.88 49.75,88.75 IC7.6 | v73.75,136.12 74.12,136.5 99.25,136.5 v102.75,133 | v104.25,89.12 104.25,92.12 83,92.12 82.38,91.5 72.25,91.5 | 72.25,91.5 66.25,91.5 65.38,92.38 64.12,92.38 63.88,92.12 v51.12,92.12 | v79.62,40.62 77.62,42.62 55.75,42.62 55.25,42.12 55.25,40.88 v70.12,40.88 | v72.25,91.38 72.25,91.5
A7  (via drill 0.61)
  Top 0.254: v72.25,137.12 66.75,131.62 CN1.18 | v100.88,137.12 100.88,114.88 98.62,112.62 v96.88,112.62 | v57.5,107 57.38,106.88 v57.38,93.6 | v81.62,87.5 81.62,42.35 83.62,40.35 83.62,32.25 IC11.37
  Bottom 0.254: IC8.37 29.62,91.5 49.62,91.5 49.75,91.38 IC7.5 | v72.25,137.12 72.62,137.5 100.5,137.5 v100.88,137.12 | v96.88,112.62 96.5,112.25 77.75,112.25 72.5,107 v57.5,107 | IC7.5 49.38,91.62 50.75,93 56.77,93 v57.38,93.6 | v81.62,87.5 78.88,90.25 64.25,90.25 63.25,91.25 49.88,91.25 IC7.5
A8  (via drill 0.61)
  Top 0.254: IC8.38 29.62,94 32.38,91.25 v32.38,90.62 32.38,87.62 35.1,84.9 35.1,43.65 34.25,42.8 34.25,22.55 34.55,22.25 34.55,13.15 40.33,7.38 v42.62,7.38 | v64.12,134.12 64.12,131.62 CN1.20 | v100,123 99.12,122.12 v99.12,116.12 | v61.25,116.38 60.38,115.5 60.38,90.38 v60,90 | IC11.59 82.5,10.12 82.6,8.22 82.6,7.72 v82.25,7.38
  Bottom 0.254: v32.38,90.62 33.12,89.88 60,89.88 | 60,89.88 63.88,89.88 65,88.75 IC7.27 | v64.12,134.12 64.25,134.25 91.12,134.25 92.38,135.5 98.75,135.5 101.38,132.88 101.38,123 v100,123 | v99.12,116.12 98.75,116.5 69.88,116.5 69.12,115.75 63.88,115.75 63.25,116.38 v61.25,116.38 | v60,90 60,89.88 | v42.62,7.38 v82.25,7.38
A9  (via drill 0.61)
  Top 0.254: v63.25,135.88 63.25,133.12 61.75,131.62 CN1.22 | v101.75,117.5 v101.75,135.25 | v68.5,117.12 68.12,116.75 68.12,89.25 65.12,86.25 IC7.26 | v75.38,34 73.12,36.25 v73.12,86 | IC11.61 84.62,10.25 84.55,10.97 84.55,23.61 v86.67,25.74 | v35.1,87.6 35.1,92.9 31.45,96.55 IC8.39
  Bottom 0.254: v63.25,135.88 63.62,136.25 72.62,136.25 73.38,137 99.75,137 101.5,135.25 v101.75,135.25 | v101.75,117.5 68.88,117.5 v68.5,117.12 | v75.38,34 77.5,31.88 94,31.88 94,29 90.74,25.74 v86.67,25.74 | v73.12,86 73,86.12 65.12,86.12 IC7.26 65,86.25 64,87.25 35.45,87.25 v35.1,87.6
A10  (via drill 0.61)
  Top 0.254: v54.5,136.25 59.12,131.62 CN1.24 | v14.62,136.62 14.38,136.38 14.38,126 21,119.38 v21,110.62 | v81.6,19.02 81.6,10.78 81.62,10.25 IC11.58 | v78.88,30.38 78.75,30.5 78.75,47.25 76.88,49.12 v76.88,74.38 | v92.05,29.4 92.05,22.62 v91.12,21.7 | v62.88,100 62,99.12 62,80 63.41,78.59 IC7.23
  Bottom 0.254: 30.5,100 29.62,99.12 IC8.40 | v62.88,100 30.5,100 | v54.5,136.25 48.25,136.25 47.5,137 15,137 v14.62,136.62 | v81.6,19.02 84.88,21.75 v91.12,21.7 | v78.88,30.38 92.05,30.38 v92.05,29.4 | v76.88,74.38 72.75,78.5 65.12,78.5 IC7.23 | v21,110.62 21,110 30.5,100.5 30.5,100
A11  (via drill 0.61)
  Top 0.254: v53.5,134.75 56.62,131.62 CN1.26 | v14.75,124.38 16.5,122.62 16.5,92.75 12,92.75 | v68.88,31.25 68.75,31.38 68.75,66 71.62,68.88 v71.62,82.75 | IC11.60 83.62,10.25 83.55,12.22 83.55,24.68 v84,25.12 | v12.62,88 12,88.62 12,92.75 | 12,92.75 12,98 13.09,99.09 IC8.1
  Bottom 0.254: v12.62,88 13.12,87.5 17.5,87.5 20.12,84.88 41.5,84.88 41.88,84.5 45.12,84.5 45.58,84.95 50.3,84.95 50.8,84.45 54.45,84.45 55.23,83.67 IC7.25 65.12,83.62 70.75,83.62 v71.62,82.75 | v53.5,134.75 23.38,134.75 22.75,135.38 18,135.38 14.38,131.75 14.38,124.38 v14.75,124.38 | v68.88,31.25 93.3,31.25 93.3,29.3 90.7,26.7 85.58,26.7 v84,25.12
A12  (via drill 0.61)
  Top 0.254: v48.62,137.12 54.12,131.62 CN1.28 | v79.75,39.25 79.75,27.75 77.12,27.75 IC11.42 | IC7.4 49.75,93.75 47.38,91.38 47.38,60.62 55,53 55,41.75 v56.12,41.75 | v10.2,101.78 v13.55,101.78
  Bottom 0.254: IC7.4 49.75,93.75 48.75,92.75 12.62,92.75 12.62,94.88 14.25,96.5 IC8.2 14.25,96.62 12.62,96.62 12.62,100.85 v13.55,101.78 | v48.62,137.12 48.25,137.5 14.25,137.5 12.5,135.75 12.5,116.25 11.38,116.25 11.12,116 11.12,102.62 10.28,101.78 v10.2,101.78 | v79.75,39.25 77.25,41.75 v56.12,41.75
A13  (via drill 0.61)
  Top 0.254: v63.08,93.62 65,91.75 65,91.38 IC7.28 | v47.12,136.12 51.62,131.62 CN1.30 | IC8.3 14.38,94.12 16,95.75 16,115.7 v15.07,116.62 | v75.75,5.38 80.5,10.12 IC11.57 | v24.38,20.38 23,21.75 23,93.5 v22.88,93.62
  Bottom 0.254: 22.88,94 27.5,94 28.62,95.12 61.62,95.12 v63.08,93.62 | 22.88,94 14.38,94 IC8.3 | v47.12,136.12 46.75,136.5 15.75,136.5 14.62,135.38 13.62,135.38 13.38,135.12 13.38,116.62 v15.07,116.62 | v75.75,5.38 39.38,5.38 v24.38,20.38 | 22.88,94 v22.88,93.62
A14  (via drill 0.61)
  Top 0.254: 76.44,31.31 77,30.75 77,28.75 IC11.41 | 76.44,31.31 72,35.75 72,38 70.75,39.25 v70.12,39.25 | 76.44,31.31 v77.88,32.75 | v89.5,133.25 91.62,135.38 98.38,135.38 v98.38,134.62 | v100,125.12 96.38,121.5 94.75,121.5 v94.75,118.38 | v43.55,116 43.25,115.7 v43.25,85.38 43.95,84.67 43.95,45.3 44.95,44.3 v44.95,41.33 | v130.5,42.38 130.5,39.12 v125,33.62
  Bottom 0.254: v43.25,85.38 20.38,85.38 14.38,91.38 IC8.4 | v70.12,39.25 47.02,39.25 v44.95,41.33 | v130.5,42.38 142,42.38 146.12,46.5 IC13.2 | v125,33.62 124.12,32.75 v77.88,32.75 | v89.5,133.25 50.88,133.25 49.25,131.62 CN1.32 | v98.38,134.62 100.88,132.12 100.88,125.12 v100,125.12 | v94.75,118.38 94.38,118 55.5,118 53,115.5 44.05,115.5 v43.55,116
A15  (via drill 0.61)
  Top 0.254: v21.88,115.25 22.5,115.88 22.5,122 26.88,126.38 v26.88,132.38 | IC11.38 82.62,32.25 82.62,37.12 v82.75,37.25 82.75,37.38 81.12,39 81.12,46.38 79.38,48.12 79.38,104.12 v79.62,104.38
  Bottom 0.254: v26.88,132.38 28.12,133.62 43.88,133.62 45.88,131.62 46.62,131.62 CN1.34 | IC8.5 14.25,89 12.12,91.12 12.12,115.25 v21.88,115.25 22,115.25 32.62,104.62 79.38,104.62 v79.62,104.38 | v82.75,37.25 98,37.25 101.75,41 134.12,41 134.5,41.38 143.5,41.38 146.12,44 IC13.3
AR0  (via drill 0.61)
  Top 0.254: v42,25.5 43.88,23.62 43.88,22.75 v44.75,21.88 | v74.38,20.12 74.38,19.75 77,19.75 IC11.50 | v59.5,21.12 54.38,21.12 54.38,22.5 IC9.14
  Bottom 0.254: v42,25.5 42,25.25 40.75,24 39.75,24 39.75,22.62 IC10.14 | v44.75,21.88 45.12,21.5 53.25,21.5 54.25,22.5 IC9.14 | v74.38,20.12 73.62,20.88 63.25,20.88 63,21.12 v59.5,21.12
AR1  (via drill 0.61)
  Top 0.254: 40.44,25.81 41.62,27 v44.25,27 | 40.44,25.81 39.75,25.12 IC10.13 | v51.5,26.62 54.25,26.62 54.25,25.12 IC9.13 | v74.38,16.62 77,16.62 IC11.53 | v45.62,11.38 45.12,11.88 45.12,20.12 42.38,22.88 42.38,23.88 40.44,25.81
  Bottom 0.254: v44.25,27 44.62,26.62 v51.5,26.62 | v74.38,16.62 73.5,15.75 65.12,15.75 63.62,14.25 63.62,11.38 v45.62,11.38
AR2  (via drill 0.61)
  Top 0.254: v52.88,34.25 52.62,34 52.62,29.38 54.25,27.75 IC9.12 | v74.38,18.88 74.38,17.75 77,17.75 IC11.52 | v72.62,20 71.75,20.88 71.75,31 v70.62,32.12
  Bottom 0.254: IC10.12 39.62,27.62 38,29.25 38,34.25 v52.88,34.25 53,34.25 53.38,33.88 56.25,33.88 57,34.62 58.88,34.62 59.25,34.25 68.5,34.25 v70.62,32.12 | v74.38,18.88 73.25,20 v72.62,20
AR3  (via drill 0.61)
  Top 0.254: v44.25,29.12 44.25,30.12 39.75,30.12 IC10.11 | v74.38,21.75 77,21.75 IC11.48 | v72.62,21.75 72.5,21.88 72.5,33.25 v70.12,35.62 | IC9.11 54.38,30.25 56,31.88 v56,36.23
  Bottom 0.254: v44.25,29.12 53,29.12 54,30.12 54.25,30.12 IC9.11 | v72.62,21.75 v74.38,21.75 | v56,36.23 56.6,35.62 v70.12,35.62
AR4  (via drill 0.61)
  Top 0.254: v58.38,31.25 61.88,31.25 61.88,30.25 IC9.8 | v74.38,23.5 74.38,23.62 77,23.62 IC11.46
  Bottom 0.254: v58.38,31.25 48.38,31.25 47.38,30.25 IC10.8 | v74.38,23.5 73.88,24 61,24 60.25,24.75 60.25,30.12 61.88,30.12 IC9.8
AR5  (via drill 0.61)
  Top 0.254: v57,28.75 61.88,28.75 61.88,27.75 IC9.7 | v73.5,27.62 73.5,15.75 77,15.75 IC11.54
  Bottom 0.254: v57,28.75 53.38,28.75 53.25,28.62 48.38,28.62 47.38,27.62 IC10.7 | v73.5,27.62 62,27.62 IC9.7
AR6  (via drill 0.61)
  Top 0.254: v57,26.12 61.88,26.12 61.88,25.12 IC9.6 | v74.38,24.75 77,24.75 IC11.45
  Bottom 0.254: v57,26.12 53.25,26.12 52.88,25.75 48,25.75 47.38,25.12 IC10.6 | v74.38,24.75 74.12,25 62,25 IC9.6
AR7  (via drill 0.61)
  Top 0.254: v74.38,32.12 74.38,25.75 77,25.75 IC11.44 | v55.12,34.75 54.38,34 54.38,32.75 IC9.10
  Bottom 0.254: IC10.10 39.75,32.75 40.75,33.75 52.12,33.75 53.12,32.75 54.25,32.75 IC9.10 | v74.38,32.12 71.75,34.75 59.5,34.75 59.12,35.12 56.75,35.12 56.38,34.75 v55.12,34.75
B  (via drill 0.61)
  Top 0.254: v101.75,13.12 101.5,13.38 101.5,14.5 101.3,14.7 100.9,14.72 99.12,14.62 IC11.10 | v67.25,13.88 65.38,15.75 65.38,44.25 62.62,47 62.62,69.5 65,69.5 66.12,70.62 66.12,79.5 67.05,80.42 v67.05,81.88 | v87.03,89.35 v87.03,94.08
  Top 0.406: R45.2 141.68,104.92 v141.68,109.5 | v113.38,97.75 113,98.12 113,105 115.89,107.89 IC21.9
  Bottom 0.254: v141.68,109.5 119.75,109.5 118.25,108 IC21.9 | v101.75,13.12 109.12,13.12 | 109.12,13.12 119.25,13.12 121,11.38 JP3.5 | v67.05,81.88 78.88,81.88 86.35,89.35 v87.03,89.35 | v67.25,13.88 69.88,11.25 107.38,11.25 109.12,13 109.12,13.12 | v87.03,94.08 87.83,94.88 112.58,94.88 113.65,95.95 113.65,97.47 v113.38,97.75
B0  (via drill 0.61)
  Top 0.254: v66.75,100.62 66.12,100 66.12,94.88 65.12,93.88 IC7.29
  Bottom 0.254: v66.75,100.62 88.5,100.62 90.25,102.38 IC4.2
B1
  Bottom 0.254: JP1.2 64.62,95.25 64.25,95.62 50.5,95.62 49.88,96.25 IC7.3
B2  (via drill 0.61)
  Top 0.254: v80.25,102.62 v82,104.38 | IC7.2 49.88,99 51.62,100.75 v51.62,102.88
  Bottom 0.254: v82,104.38 85.62,104.38 85.88,104.12 103.38,104.12 103.88,103.62 104,103.62 104,101.75 105.12,100.62 106.62,100.62 106.62,106.38 103,110 IC4.10 | v80.25,102.62 80,102.88 v51.62,102.88
BEEPER  (via drill 0.61)
  Top 0.254: v149.12,69.88 149.12,54.5 150.38,53.25 v150.38,32.5 | v106.25,27.23 106.25,20.12 105.75,19.62 99.12,19.62 IC11.15 | v157.62,76.5 157.62,76.76
  Top 0.406: R31.1 157.62,76.76 R33.1
  Bottom 0.254: v157.62,76.5 151,69.88 v149.12,69.88 | v150.38,32.5 148.25,30.38 135.38,30.38 135.25,30.5 112.12,30.5 108.85,27.23 v106.25,27.23
BR  (via drill 0.61)
  Top 0.254: 125.88,90.12 IC21.1 | 125.88,92.62 IC21.2 125.88,92.75 | 125.88,95.12 IC21.3 125.75,95.25 | 118.25,92.75 IC21.15 | 118.25,95.12 IC21.14 | 118.25,97.62 IC21.13 118.25,97.75 | 118.25,95.25 IC21.14 | 118.25,100.25 IC21.12 | v101.88,22.75 99.12,22.75 IC11.18 | v110,22.75 110,73 110.38,73.38 110.38,75.5 110.12,75.75 110.12,90.75 v109.88,91 | 118.38,95.25 IC21.14
  Top 0.406: 125.88,92.62 125.88,90.12 | 125.88,92.75 125.88,95.12 | 118.25,95.12 118.25,92.75 | 118.25,95.25 118.25,97.62 | 118.25,97.75 118.25,100.25 | 118.38,95.25 125.75,95.25
  Bottom 0.254: v110,22.75 v101.88,22.75 | v109.88,91 111.5,92.62 118.12,92.62 IC21.15
CA  (via drill 0.61)
  Top 0.254: v146.88,58 146.88,67.25 145.25,68.88 R35.2 | v169.88,55.5 170.25,55.12 v170.25,43.62 | v185.88,42.75 185.88,39.38 IC12.4
  Bottom 0.254: v146.88,58 149.38,55.5 v169.88,55.5 | v170.25,43.62 171.38,42.75 v185.88,42.75
CB  (via drill 0.61)
  Top 0.254: v163.5,68 162.12,68 162.12,68.75 R32.2 | v176.62,41.38 175.55,42.45 175.55,48.9 174.85,49.6 173.75,49.6 173.75,60.25 170.62,63.38 v170.62,68
  Top 0.406: R34.2 R32.2
  Bottom 0.254: v176.62,41.38 181.38,41.38 183.38,39.38 IC12.3 | v163.5,68 v170.62,68
CC  (via drill 0.61)
  Top 0.254: 172.88,68.88 R30.2 172.77,62.23 174.93,60.08 v174.93,51.5
  Bottom 0.254: v174.93,51.5 185,51.5 187,53.5 187,56.25 185.12,56.25 183.5,54.62 IC12.38
CLC2  (via drill 0.61)
  Top 0.254: IC16.11 185.79,64.81 186.75,63.85 192.85,63.85 200.12,56.58 200.12,52.02 v200.78,51.38
  Bottom 0.254: IC12.22 224,54.5 220.88,51.38 v200.78,51.38
CLK  (via drill 0.61)
  Top 0.254: v17.25,58.12 17.25,74.75 17,75 13,75 12,76 12,86 12.39,86.39 IC8.6 | IC11.31 89.5,32.25 89.5,36.15 88.85,36.8 88.85,52.27 v87.25,53.88
  Bottom 0.254: v87.25,53.88 40.25,53.88 39.48,54.65 22.85,54.65 21.9,53.7 20.45,53.7 19,55.15 19,57 17.88,58.12 v17.25,58.12
D0  (via drill 0.61)
  Top 0.254: v48.25,63 48.25,62.38 56.54,54.09 R22.1 | 56.5,43.38 R22.1 | v145.25,52.88 148,50.12 148,46.25 146.88,45.12 144.25,45.12 v144.25,43.38 | v57.5,44.75 56.38,43.62 R22.1
  Bottom 0.254: v48.25,63 44.12,67.12 15.38,67.12 14.38,66.12 IC8.14 | v145.25,52.88 144.88,53.25 140.5,53.25 138.5,51.25 IC6.2 | v144.25,43.38 142.75,41.88 134.25,41.88 133.88,41.5 102.75,41.5 100.25,44 58.25,44 v57.5,44.75
D1  (via drill 0.61)
  Top 0.254: v50,44.75 51.5,43.25 R21.1 | v149.5,52.88 149.12,52.5 149.12,34.62 147.12,32.62 v144.88,32.62 | v113,35 110.88,37.12 v110.88,42.38
  Bottom 0.254: IC8.15 14.25,63.5 12.62,63.5 12.62,57.2 16.2,57.2 17.35,56.05 17.35,53.52 23.62,47.25 47.5,47.25 v50,44.75 50.12,44.75 51.88,46.5 73.62,46.5 75.25,44.88 108.38,44.88 v110.88,42.38 | v149.5,52.88 148.62,53.75 138.5,53.75 IC6.3 | v144.88,32.62 142.5,35 v113,35
D2  (via drill 0.61)
  Top 0.254: 45.62,45.62 45.62,44.12 46.5,43.25 R20.1 | v153,54.25 155.62,51.62 155.62,31 v152.88,28.25 | v143.88,28.25 141.25,30.88 v141.25,31.88 | v77.12,33.75 74,36.88 v74,44.88 | 45.62,45.62 v52.25,45.62 | v45.23,71.47 45.23,46.02 45.62,45.62
  Bottom 0.254: IC8.12 14.38,71.25 15.57,72.45 44.25,72.45 v45.23,71.47 | v153,54.25 140.5,54.25 138.5,56.25 IC6.4 | v143.88,28.25 v152.88,28.25 | v141.25,31.88 138.62,34.5 116.25,34.5 115.5,33.75 v77.12,33.75 | v74,44.88 73.25,45.62 v52.25,45.62
D3  (via drill 0.61)
  Top 0.254: v37.62,79.95 37.62,51.25 | 37.62,51.25 37.62,47.12 41.5,43.25 R19.1 | v150,56.38 151.25,55.12 v151.25,49.62 | v37.75,51.25 37.62,51.25 | v118.62,46.12 v118.62,49.5
  Bottom 0.254: IC8.8 14.38,81.25 15.38,80.25 37.33,80.25 v37.62,79.95 | v150,56.38 147.5,58.88 138.5,58.88 IC6.5 | v151.25,49.62 149.25,47.62 144.88,47.62 142.25,45 128.75,45 127.25,46.5 127.25,52.25 120,52.25 119.55,51.8 119.55,50.42 v118.62,49.5 | v37.75,51.25 38,51.5 104.62,51.5 113.72,42.4 116.1,42.4 118.62,44.92 v118.62,46.12
D4  (via drill 0.61)
  Top 0.254: v106,39.62 106,42.62 105.38,43.25 R18.1 105.25,43.38 105.25,47.25 v104.5,48 | v138.62,40 141.38,42.75 141.38,58.5 138.5,61.38 IC6.6 | v22,81.12 22.12,81 v22.12,51.25
  Bottom 0.254: v106,39.62 106.38,40 v138.62,40 | v22,81.12 17,81.12 14.38,83.75 IC8.7 | v22.12,51.25 25.62,47.75 50.62,47.75 50.88,48 v104.5,48
D5  (via drill 0.61)
  Top 0.254: v100.38,38.38 100.38,43.25 R17.1 100.38,43.38 100.38,52.88 v94.88,58.38 | v139.62,38.12 140.62,39.12 141.88,39.12 141.88,60.5 138.5,63.88 IC6.7 | v20.25,65 17.75,67.5 17.75,75.38 14.38,78.75 IC8.9
  Bottom 0.254: v100.38,38.38 100.62,38.12 v139.62,38.12 | v20.25,65 22.75,62.5 45.75,62.5 46.12,62.12 51.25,62.12 52,62.88 64,62.88 64.88,62 91.25,62 v94.88,58.38
D6  (via drill 0.61)
  Top 0.254: v60.38,72.25 60.38,44.38 61.38,43.38 R16.1 61.38,43.25 61.38,36.62 v61.25,36.5 | v150,62 156.62,55.38 v156.62,28.25 | v111.38,34.83 111.38,29.88 v115.9,25.35
  Bottom 0.254: v60.38,72.25 55.38,77.25 15.38,77.25 14.38,76.25 IC8.10 | v150,62 148.75,62 144.88,65.88 139,65.88 138.5,66.38 IC6.8 | v156.62,28.25 155.62,27.25 140.88,27.25 138.97,25.35 v115.9,25.35 | v61.25,36.5 70.75,36.5 72.38,34.88 111.33,34.88 v111.38,34.83
D7  (via drill 0.61)
  Top 0.254: v95.5,36.38 95.5,43.25 R15.1 | v138.12,36.75 137.75,37.12 137.75,47.25 136.12,48.88 136.12,66.38 138.38,68.62 138.38,69 IC6.9 | v31.75,45.12 32,44.88 v32,41.38
  Bottom 0.254: v138.12,36.75 95.88,36.75 v95.5,36.38 82.38,36.38 80.88,37.88 39.12,37.88 35.62,41.38 v32,41.38 | IC8.13 14.25,68.5 12.12,66.38 12.12,52.88 12.85,52.15 16.85,52.15 23.88,45.12 v31.75,45.12
DB0  (via drill 0.61)  (1 unrouted)
  Top 0.254: v119.38,53.75 IC2.18 | v142.75,47.12 v142.75,51.88 | v28.75,117.12 28.75,116.38 28,115.62 R12.2 | v61.75,59.62 61.25,60.12 v61.25,66.75 | 54.12,126.5 53.42,125.8 v53.42,118.03 | v47.88,105.5 48,105.38 48,98 48.4,97.6 51.62,97.6 | 51.62,97.6 v51.62,98.75 | IC7.13 48.3,72.46 48.3,86.9 48.85,87.45 50.7,87.45 52,88.75 52,96 51.62,96.38 51.62,97.6
  Bottom 0.254: v119.38,53.75 120.38,52.75 128,52.75 | 128,52.75 129,53.75 130.75,53.75 IC6.18 | v142.75,51.88 143.12,51.5 158.88,51.5 160.75,53.38 171.75,53.38 171.88,53.25 177.25,53.25 177.62,52.88 184.25,52.88 185.88,54.5 IC12.37 | v142.75,47.12 141.38,45.75 129,45.75 128,46.75 128,52.75 | 39.62,117.12 52.52,117.12 v53.42,118.03 | 39.62,117.12 v28.75,117.12 | v51.62,98.75 63.15,98.75 64.6,100.2 65.6,100.2 66.05,99.75 67.12,99.75 67.5,100.12 93,100.12 95.25,102.38 IC4.4 | 39.62,117.12 39.62,105.5 v47.88,105.5 | v61.75,59.62 63.88,57.5 110.5,57.5 114.25,53.75 IC2.18 | v61.25,66.75 57.12,70.88 49.88,70.88 IC7.13
DB1  (via drill 0.61)
  Top 0.254: v119.38,58.75 114.38,58.75 IC2.16 | v187.12,47.38 187.12,53.25 188.38,54.5 IC12.36 | v136.12,68.75 132.25,72.62 126,72.62 v126,57.5 | 37.75,115.62 R11.2 37.64,118.21 v37.45,118.4 | 54.25,98.75 v55.12,97.88 | 54.25,98.75 54.25,113.05 52.02,115.28 v52.02,118.62 52.02,126.22 CN1.29 | IC7.14 49.88,68.38 51.5,66.75 51.5,60.83 54.12,60.83 54.12,98.75 54.25,98.75 | v108.12,62.5 107.62,63 v107.62,83.75 | v105.03,86.35 101.5,89.88 101.5,98.88 98,102.38 IC4.5 | v172,59.88 172,53.6 172.8,52.8 172.8,48.6 174.5,48.6 v174.5,46.5
  Bottom 0.254: v119.38,58.75 120.75,57.38 126,57.38 | 126,57.38 129.75,57.38 130.75,56.38 IC6.17 | v187.12,47.38 186.25,46.5 v174.5,46.5 | v172,59.88 144.5,59.88 139,65.38 137.38,65.38 136.62,66.12 136.62,66.88 136.88,67.12 136.88,68.38 136.5,68.38 v136.12,68.75 | v126,57.5 126,57.38 | v52.02,118.62 37.67,118.62 v37.45,118.4 | IC4.5 95.12,99.62 67.75,99.62 66,97.88 v55.12,97.88 | v108.12,62.5 110.62,62.5 114.25,58.88 IC2.16 | v105.03,86.35 v107.62,83.75
DB2  (via drill 0.61)
  Top 0.254: v48.12,122.62 48.12,116.38 47.38,115.62 R10.2 | v94.88,113.12 97.88,110.12 IC4.12 | 47.38,115.5 R10.2 | v119.5,60.12 115.75,63.88 114.38,63.88 IC2.14 | v188,48.25 188,51.5 191,54.5 IC12.35 | v158.5,52.38 v161.25,49.62 | v144,49.62 v144,52.38 | v55,123 55,124.92 CN1.25 | R10.2 47.29,113.81 v47.23,113.75 46.45,112.97 46.45,69.4 v46.3,69.25
  Bottom 0.254: v48.12,122.62 48.5,123 v55,123 | v94.88,113.12 65.88,113.12 65.25,113.75 v47.23,113.75 | v119.5,60.12 129.5,60.12 130.75,58.88 IC6.16 130.88,58.75 132.5,58.75 133,58.25 133,53.5 132,52.5 129.25,52.5 128.7,51.95 128.7,46.8 129.25,46.25 140.62,46.25 v144,49.62 | v188,48.25 176.3,48.35 162.62,48.25 v161.25,49.62 | v158.5,52.38 158.12,52 144.38,52 v144,52.38 | IC2.14 114.25,64 113.88,64.38 65.12,64.38 63.62,65.88 49.88,65.88 IC7.15 49.66,65.89 v46.3,69.25
DB3  (via drill 0.61)
  Top 0.254: 113.44,65.31 113.75,65 115.38,65 117.5,62.88 v123.75,62.88 | 113.44,65.31 112.62,66.12 112.62,67.25 114.25,68.88 IC2.12 | v190.5,49.62 190.5,51.5 193.5,54.5 IC12.34 | v160.75,51.38 v162.5,49.62 | v56,65 56,115.5 R9.2 55.88,115.62 55.88,119.5 v55,120.38 | v27.88,120.38 27.88,127.88 40.5,127.88 44.12,131.5 CN1.36 | 113.44,65.31 111.75,63.62 v111.75,63.5 | v134.85,50.12 134,50.98 134,60 132.62,61.38 IC6.15
  Bottom 0.254: v123.75,62.88 125.12,61.5 130.75,61.5 IC6.15 | v190.5,49.62 190.12,50 162.88,50 v162.5,49.62 | v160.75,51.38 160.38,51 140.25,51 139.38,50.12 v134.85,50.12 | v56,65 57.62,63.38 65,63.38 IC7.17 65.12,63.38 111.62,63.38 v111.75,63.5 | v55,120.38 v27.88,120.38
DB4  (via drill 0.61)
  Top 0.254: v44.12,124 44.12,126.5 CN1.35 | 64.5,115.62 R8.2 | IC12.33 193.12,51.62 v193.12,49.62 | v177.38,49.12 176,50.5 v176,54.12 | v136,67.5 132.5,64 130.88,64 IC6.14 | v116.25,65.38 116.12,65.5 116.12,68.25 116.75,68.88 121.88,68.88 IC2.9 | v65,112.75 65,115.12 64.62,115.5 R8.2 | v68.25,67.5 69.88,69.12 69.88,111.62 v70.5,112.25 | v62.38,124 64.59,121.78 R8.2
  Bottom 0.254: v44.12,124 44.5,124.38 62,124.38 v62.38,124 | IC2.9 122,68.88 123.38,67.5 131.88,67.5 132.5,66.88 132.5,64 130.88,64 IC6.14 | v193.12,49.62 192.25,48.75 190.12,48.75 189.75,49.12 v177.38,49.12 | v176,54.12 170.75,59.38 142.5,59.38 139,62.88 137.25,62.88 136,64.12 v136,67.5 | 68.25,64.88 113.25,64.88 113.75,65.38 v116.25,65.38 | 68.25,64.88 66.12,64.88 65.12,65.88 IC7.18 | v65,112.75 65.5,112.25 v70.5,112.25 | 68.25,64.88 v68.25,67.5
DB5  (via drill 0.61)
